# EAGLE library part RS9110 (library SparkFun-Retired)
Redpine WiFi module
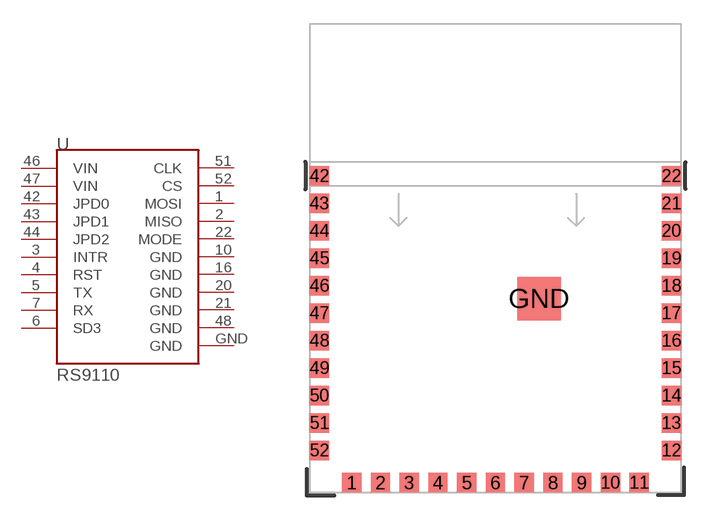
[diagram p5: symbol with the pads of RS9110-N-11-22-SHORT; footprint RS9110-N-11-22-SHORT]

Designator prefix U

## RS9110 (PROD_ID: IC-10622)  [RS9110-N-11-22-SHORT]
1  MOSI
2  MISO
3  INTR
4  RST
5  TX
6  SD3
7  RX
10  GND
16  GND
20  GND
21  GND
22  MODE
42  JPD0
43  JPD1
44  JPD2
46  VIN
47  VIN
48  GND
51  CLK
52  CS
GND  GND

## Footprint RS9110-N-11-22-SHORT (pad centres in mm)
Redpine WiFi module: short FP (doesn't include the NC pads around the antenna)
smd 1.2 x 1.2: 1 -8.9,-13.9; 2 -7.12,-13.9; 3 -5.34,-13.9; 4 -3.56,-13.9; 5 -1.78,-13.9; 6 0,-13.9; 7 1.78,-13.9; 8 3.56,-13.9; 9 5.34,-13.9; 10 7.12,-13.9; 11 8.9,-13.9; 12 10.9,-11.9; 13 10.9,-10.2; 14 10.9,-8.5; 15 10.9,-6.8; 16 10.9,-5.1; 17 10.9,-3.4; 18 10.9,-1.7; 19 10.9,0; 20 10.9,1.7; 21 10.9,3.4; 22 10.9,5.1; 42 -10.9,5.1; 43 -10.9,3.4; 44 -10.9,1.7; 45 -10.9,0; 46 -10.9,-1.7; 47 -10.9,-3.4; 48 -10.9,-5.1; 49 -10.9,-6.8; 50 -10.9,-8.5; 51 -10.9,-10.2; 52 -10.9,-11.9
smd 2.7 x 2.7: GND 2.7,-2.5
